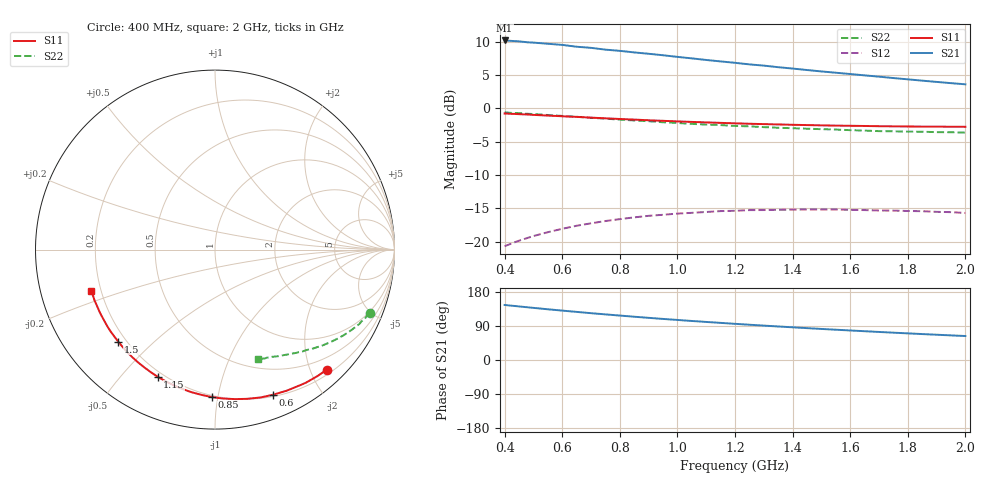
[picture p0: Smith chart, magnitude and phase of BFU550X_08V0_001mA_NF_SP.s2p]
! Filename:  P:\Prog\Test\Noise\ATS_data\Testdata_Net\BFU550X no attenuator noise\BFU550X_APG2013_44_C05_08p0V_001mA_NF_CM01_D.sf
! Date/Time: Fri 26/Jul/2013 14:37:12
! BFU550X_APG2013_44_C05_08p0V_1to10mA_NF_CM01_Bias1_R.sf
! Noise Parameter Data File
! BFU550X_APG2013_44_C05_08p0V_1to10mA_NF_CM01
! Date/time: Wed Jul 24 17:16:38 2013
! freq range =  0.4000 to  2.0000 GHz, 37 points
! bias range =  1.0000 to 10.0000 mA, 5 points
! bias supplies used: 1 1 0 0 0 0
! VAR bias_mode= 1  ! Specify V_out, I_out
! VAR bias_var = 1  ! Bias variable = I_out
! VAR V_out= 8.000000
! VAR I_out= 1.000000
! VAR V_in= 0.774900
! VAR I_in= 0.010401
! Device data file deembeded for feedlines and parallel
! Original file: \BFU550X no attenuator noise\BFU550X_APG2013_44_C05_08p0V_001mA_NF_CM01_R.sf
! Feed-files: PR005V01_100713_Feed1.s2p, PR005V01_100713_Feed2.s2p
! Parallel-file: PR005V01_100713_Par.s2p
# MHz S MA R 50
!  Freq-MHz  S11-mag  S11-arg  S21-mag  S21-arg  S12-mag  S12-arg  S22-mag  S22-arg
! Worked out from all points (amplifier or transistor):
!   37 points, 400 MHz to 2 GHz, reference 50 ohm
!   highest |S21| = 10.2 dB at 400 MHz (marker M1)
!   |S21| within 3 dB of that: start of sweep to 1.117 GHz
!   unconditionally stable (mu >= 1): nowhere
!   at 500 MHz: K = 0.13, MSG = 14.5 dB, |S12| = -19.2 dB
!   at 1.1 GHz: K = 0.27, MSG = 11.4 dB, |S12| = -15.6 dB
!   at 2 GHz: K = 0.49, MSG = 9.6 dB, |S12| = -15.7 dB
!   lowest NFmin = 0.55 dB at 460 MHz
!   S11 on the Smith chart (normalised r, x): 400 MHz: 0.28, -2.26; 600 MHz: 0.22, -1.45; 850 MHz: 0.19, -0.96; 1.15 GHz: 0.18, -0.63; 1.5 GHz: 0.17, -0.39; 2 GHz: 0.16, -0.16
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400  0.9135 -47.1  3.224 145.2  0.09244 60.4  0.9327 -22.4
440  0.9054 -51.5  3.187 142.1  0.09984 57.9  0.9216 -24.2
480  0.8978 -55.7  3.123 139.1  0.1066 55.3  0.9085 -26.1
500  0.892 -57.9  3.107 137.6  0.1101 54.0  0.9055 -27.1
550  0.8816 -63.1  3.045 133.8  0.1176 51.0  0.8899 -29.4
600  0.8708 -68.2  2.987 130.3  0.1248 48.1  0.876 -31.5
650  0.8618 -73.0  2.893 127.0  0.1315 45.3  0.8629 -33.4
700  0.8505 -77.8  2.838 123.5  0.1372 42.6  0.8481 -35.4
750  0.8408 -82.2  2.751 120.4  0.1427 40.1  0.8355 -37.1
800  0.8311 -86.8  2.696 117.3  0.1474 37.6  0.8219 -39.0
850  0.8223 -91.1  2.623 114.2  0.152 35.2  0.8101 -40.6
900  0.8128 -95.4  2.562 111.2  0.1561 32.9  0.7995 -42.2
950  0.8051 -99.4  2.498 108.4  0.1589 30.6  0.7852 -43.9
1050  0.79 -107.0  2.366 103.0  0.1644 26.6  0.7636 -46.8
1150  0.7771 -114.2  2.245 98.0  0.1693 22.7  0.7481 -49.3
1200  0.7707 -117.8  2.192 95.4  0.1703 20.8  0.7372 -50.8
1350  0.7562 -127.5  2.032 88.5  0.1732 15.8  0.7141 -54.5
1500  0.7442 -136.4  1.889 82.0  0.1742 11.1  0.6969 -57.9
1600  0.739 -142.0  1.806 77.9  0.1731 8.2  0.6852 -60.3
1750  0.7318 -149.8  1.685 72.1  0.1709 4.4  0.6719 -63.4
1850  0.7284 -154.6  1.611 68.4  0.1691 2.0  0.667 -65.4
2000  0.7262 -161.6  1.512 63.3  0.164 -1.1  0.6568 -68.5
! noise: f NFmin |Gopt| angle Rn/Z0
400  0.6478  0.6418  27.95  0.3267
460  0.5491  0.6446  37.75  0.2866
600  0.7086  0.6627  45.77  0.3527
800  0.7344  0.6597  63.02  0.2887
1000  0.7874  0.6241  76.94  0.2718
1200  0.8851  0.648  92.88  0.2185
1400  0.9818  0.6727  106.1  0.2138
1600  0.7862  0.6011  122.4  0.1179
1800  0.8013  0.627  136  0.0868
2000  1.073  0.7091  143.8  0.0785
